| ussxh8g16bc.ibs * IBIS 4.2 Model
| 8Gb DDR3L SDRAM
| This Model is valid for Commercial Temperature Range 0C<=Tc<=85C
| Valid for DDR3L-1066/1333/1600/1866 operation
[IBIS Ver]   4.2
[File Name]   ussxh8g16bc.ibs
[Date]   10/19/2018
[File Rev]   2.0
| COMPONENT: SCB13(15)H8G162BF (96-Ball FBGA, x16, 7.5mm X 13.5mm)
[Component]   SCB13(15)H8G162BF
[Manufacturer]  UniIC Semiconductors Corp.
[Package]
|   typ   min   max
R_pkg   454.1m   301.3m   636.7m
L_pkg   1.754nH   1.047nH   2.886nH
C_pkg   0.475pF   0.334pF   0.777pF
[Pin]   signal_name  model_name   R_pin   L_pin   C_pin
A1   VDDQ   POWER
A2   DQ13   DQ
A3   DQ15   DQ
A7   DQ12   DQ
A8   VDDQ   POWER
A9   VSS   GND
B1   VSSQ   GND
B2   VDD   POWER
B3   VSS   GND
B7   UDQS#   DQS
B8   DQ14   DQ
B9   VSSQ   GND
C1   VDDQ   POWER
C2   DQ11   DQ
C3   DQ9   DQ
C7   UDQS   DQS
C8   DQ10   DQ
C9   VDDQ   POWER
D1   VSSQ   GND
D2   VDDQ   POWER
D3   UDM   DM
D7   DQ8   DQ
D8   VSSQ   GND
D9   VDD   POWER
E1   VSS   GND
E2   VSSQ   GND
E3   DQ0   DQ
E7   LDM   DM
E8   VSSQ   GND
E9   VDDQ   POWER
F1   VDDQ   POWER
F2   DQ2   DQ
F3   LDQS   DQS
F7   DQ1   DQ
F8   DQ3   DQ
F9   VSSQ   GND
G1   VSSQ   GND
G2   DQ6   DQ
G3   LDQS#   DQS
G7   VDD   POWER
G8   VSS   GND
G9   VSSQ   GND
H1   VREFDQ   POWER
H2   VDDQ   POWER
H3   DQ4   DQ
H7   DQ7   DQ
H8   DQ5   DQ
H9   VDDQ   POWER
J1   NC   NC
J2   VSS   GND
J3   RAS#   INPUT
J7   CK   CLKIN
J8   VSS   GND
J9   NC   NC
K1   ODT   INPUT
K2   VDD   POWER
K3   CAS#   INPUT
K7   CK#   CLKIN
K8   VDD   POWER
K9   CKE   INPUT
L1   NC   NC
L2   CS#   INPUT
L3   WE#   INPUT
L7   A10   INPUT
L8   ZQ   NC
L9   NC   NC
M1   VSS   GND
M2   BA0   INPUT
M3   BA2   INPUT
M7   A15   INPUT
M8   VREFCA   POWER
M9   VSS   GND
N1   VDD   POWER
N2   A3   INPUT
N3   A0   INPUT
N7   A12   INPUT
N8   BA1   INPUT
N9   VDD   POWER
P1   VSS   GND
P2   A5   INPUT
P3   A2   INPUT
P7   A1   INPUT
P8   A4   INPUT
P9   VSS   GND
R1   VDD   POWER
R2   A7   INPUT
R3   A9   INPUT
R7   A11   INPUT
R8   A6   INPUT
R9   VDD   POWER
T1   VSS   GND
T2   RESET#   RESET
T3   A13   INPUT
T7   A14   INPUT
T8   A8   INPUT
T9   VSS   GND
|***********************PIN MAPPING*****************************************
[Pin Mapping] pulldown_ref pullup_ref gnd_clamp_ref power_clamp_ref ext_ref
A1   NC   VDDQ
A2   VSS   VDDQ   VSS   VDDQ
A3   VSS   VDDQ   VSS   VDDQ
A7   VSS   VDDQ   VSS   VDDQ
A8   NC   VDDQ
A9   VSS   NC
B1   VSS   NC
B2   NC   VDD
B3   VSS   NC
B7   VSS   VDDQ   VSS   VDDQ
B8   VSS   VDDQ   VSS   VDDQ
B9   VSS   NC
C1   NC   VDDQ
C2   VSS   VDDQ   VSS   VDDQ
C3   VSS   VDDQ   VSS   VDDQ
C7   VSS   VDDQ   VSS   VDDQ
C8   VSS   VDDQ   VSS   VDDQ
C9   NC   VDDQ
D1   VSS   NC
D2   NC   VDDQ
D3   NC   NC   VSS   VDDQ
D7   VSS   VDDQ   VSS   VDDQ
D8   VSS   NC
D9   NC   VDD
E1   VSS   NC
E2   VSS   NC
E3   VSS   VDDQ   VSS   VDDQ
E7   NC   NC   VSS   VDDQ
E8   VSS   NC
E9   NC   VDDQ
F1   NC   VDDQ
F2   VSS   VDDQ   VSS   VDDQ
F3   VSS   VDDQ   VSS   VDDQ
F7   VSS   VDDQ   VSS   VDDQ
F8   VSS   VDDQ   VSS   VDDQ
F9   VSS   NC
G1   VSS   NC
G2   VSS   VDDQ   VSS   VDDQ
G3   VSS   VDDQ   VSS   VDDQ
G7   NC   VDD
G8   VSS   NC
G9   VSS   NC
H1   NC   VREFDQ
H2   NC   VDDQ
H3   VSS   VDDQ   VSS   VDDQ
H7   VSS   VDDQ   VSS   VDDQ
H8   VSS   VDDQ   VSS   VDDQ
H9   NC   VDDQ
J1   NC   NC
J2   VSSL   NC
J3   NC   NC   VSS   VDD
J7   NC   NC   VSS   VDD
J8   VSS   NC
J9   NC   NC
K1   NC   NC   VSS   VDD
K2   NC   VDDL
K3   NC   NC   VSS   VDD
K7   NC   NC   VSS   VDD
K8   NC   VDD
K9   NC   NC   VSS   VDD
L1   NC   NC
L2   NC   NC   VSS   VDD
L3   NC   NC   VSS   VDD
L7   NC   NC   VSS   VDD
L8   NC   NC
L9   NC   NC
M1   VSS   NC
M2   NC   NC   VSS   VDD
M3   NC   NC   VSS   VDD
M7   NC   NC
M8   NC   VREFCA
M9   VSS   NC
N1   NC   VDD
N2   NC   NC   VSS   VDD
N3   NC   NC   VSS   VDD
N7   NC   NC   VSS   VDD
N8   NC   NC   VSS   VDD
N9   NC   VDD
P1   VSS   NC
P2   NC   NC   VSS   VDD
P3   NC   NC   VSS   VDD
P7   NC   NC   VSS   VDD
P8   NC   NC   VSS   VDD
P9   VSS   NC
R1   NC   VDD
R2   NC   NC   VSS   VDD
R3   NC   NC   VSS   VDD
R7   NC   NC   VSS   VDD
R8   NC   NC   VSS   VDD
R9   NC   VDD
T1   VSS   NC
T2   NC   NC   VSS   VDD
T3   NC   NC   VSS   VDD
T7   NC   NC   VSS   VDD
T8   NC   NC   VSS   VDD
T9   VSS   NC
|**********************DIFF PIN*********************************************
[Diff_pin]   inv_pin   vdiff   tdelay_typ   tdelay_min   tdelay_max
   C7   B7   0.320V   0ns   NA   NA
   F3   G3   0.320V   0ns   NA   NA
   J7   K7   0.320V   0ns   NA   NA
|   Model Selector
[Model Selector] DQ
DQ_34   34 Ohm Data I/O with no ODT, 800-2133Mbps
DQ_40   40 Ohm Data I/O with no ODT, 800-2133Mbps
DQ_IN_ODT20   Data Input with 20ohm ODT, 800-2133Mbps
DQ_IN_ODT30   Data Input with 30ohm ODT, 800-2133Mbps
DQ_IN_ODT40   Data Input with 40ohm ODT, 800-2133Mbps
DQ_IN_ODT60   Data Input with 60ohm ODT, 800-2133Mbps
DQ_IN_ODT120  Data Input with 120ohm ODT, 800-2133Mbps
[Model Selector] DQS
DQS_34   34 Ohm Data Strobe I/O with no ODT, 800-2133Mbps
DQS_40   40 Ohm Data Strobe I/O with no ODT, 800-2133Mbps
DQS_IN_ODT20  Data Strobe Input with 20ohm ODT, 800-2133Mbps
DQS_IN_ODT30  Data Strobe Input with 30ohm ODT, 800-2133Mbps
DQS_IN_ODT40  Data Strobe Input with 40ohm ODT, 800-2133Mbps
DQS_IN_ODT60  Data Strobe Input with 60ohm ODT, 800-2133Mbps
DQS_IN_ODT120 Data Strobe Input with 120ohm ODT, 800-2133Mbps
[Model Selector] DM
DM_INPUT   DM Input Model with no ODT, 800-2133Mbps
DM_ODT20   DM Input Model with 20ohm ODT, 800-2133Mbps
DM_ODT30   DM Input Model with 30ohm ODT, 800-2133Mbps
DM_ODT40   DM Input Model with 40ohm ODT, 800-2133Mbps
DM_ODT60   DM Input Model with 60ohm ODT, 800-2133Mbps
DM_ODT120   DM Input Model with 120ohm ODT, 800-2133Mbps
[Model Selector] DM_TDQS
DM_INPUT   DM Input Model with no ODT, 800-2133Mbps
DM_ODT20   DM Input Model with 20ohm ODT, 800-2133Mbps
DM_ODT30   DM Input Model with 30ohm ODT, 800-2133Mbps
DM_ODT40   DM Input Model with 40ohm ODT, 800-2133Mbps
DM_ODT60   DM Input Model with 60ohm ODT, 800-2133Mbps
DM_ODT120   DM Input Model with 120ohm ODT, 800-2133Mbps
TDQS_ODT20   TDQS Terminator Model with 20ohm ODT, 800-2133Mbps
TDQS_ODT30   TDQS Terminator Model with 30ohm ODT, 800-2133Mbps
TDQS_ODT40   TDQS Terminator Model with 40ohm ODT, 800-2133Mbps
TDQS_ODT60   TDQS Terminator Model with 60ohm ODT, 800-2133Mbps
TDQS_ODT120   TDQS Terminator Model with 120ohm ODT, 800-2133Mbps
[Model Selector] NF_TDQS#
NF_INPUT   Non-Functioning Terminator Model
TDQS_ODT20   TDQS Terminator Model with 20ohm ODT, 800-2133Mbps
TDQS_ODT30   TDQS Terminator Model with 30ohm ODT, 800-2133Mbps
TDQS_ODT40   TDQS Terminator Model with 40ohm ODT, 800-2133Mbps
TDQS_ODT60   TDQS Terminator Model with 60ohm ODT, 800-2133Mbps
TDQS_ODT120   TDQS Terminator Model with 120ohm ODT, 800-2133Mbps
| Sparse Matrix Package Model for B5116ECMDXG_96ball_pkg (x16)
[Define Package Model]  KTC_8G3D_x16_RDL_DDP_PKG
[Manufacturer]  UniIC Semiconductors Corp.
[OEM]  UniIC
[Description]  None
[Number Of Pins]  51
[Pin Numbers]
|Pin Num   Terminal Name
N3   | A0:A0_DIEtop_78
P7   | A1:A1_DIEtop_83
P3   | A2:A2_DIEtop_82
N2   | A3:A3_DIEtop_74
P8   | A4:A4_DIEtop_79
P2   | A5:A5_DIEtop_80
R8   | A6:A6_DIEtop_81
R2   | A7:A7_DIEtop_84
T8   | A8:A8_DIEtop_85
R3   | A9:A9_DIEtop_86
L7   | A10:A10_DIEtop_65
R7   | A11:A11_DIEtop_87
N7   | A12:A12_DIEtop_75
T3   | A13:A13_DIEtop_88
T7   | A14:A14_DIEtop_89
M7   | A15:A15_DIEtop_73
M2   | BA0:BA0_DIEtop_70
N8   | BA1:BA1_DIEtop_71
M3   | BA2:BA2_DIEtop_72
K3   | CASB:CASB_DIEtop_62
J7   | CK:CK_DIEtop_57
K7   | CKB:CKB_DIEtop_58
K9   | CKE:CKE_DIEtop_59
L2   | CSB:CSB_DIEtop_63
E7   | DML:DML_DIEbot_30
D3   | DMU:DMU_DIEtop_30
E3   | DQL0:DQL0_DIEbot_32
F7   | DQL1:DQL1_DIEbot_34
F2   | DQL2:DQL2_DIEbot_36
F8   | DQL3:DQL3_DIEbot_38
H3   | DQL4:DQL4_DIEbot_47
H8   | DQL5:DQL5_DIEbot_45
G2   | DQL6:DQL6_DIEbot_43
H7   | DQL7:DQL7_DIEbot_49
F3   | DQSL:DQSL_DIEbot_40
G3   | DQSLB:DQSLB_DIEbot_41
C7   | DQSU:DQSU_DIEtop_40
B7   | DQSUB:DQSUB_DIEtop_41
D7   | DQU0:DQU0_DIEtop_32
C3   | DQU1:DQU1_DIEtop_34
C8   | DQU2:DQU2_DIEtop_36
C2   | DQU3:DQU3_DIEtop_38
A7   | DQU4:DQU4_DIEtop_47
A2   | DQU5:DQU5_DIEtop_45
B8   | DQU6:DQU6_DIEtop_43
A3   | DQU7:DQU7_DIEtop_49
J1   | ODT:ODT_DIEtop_61
J3   | RASB:RASB_DIEtop_60
T2   | RESETB:RESETB_DIEtop_92
L3   | WEB:WEB_DIEtop_64
L8   | ZQ:ZQ_DIEtop_69
[Model Data]
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[End Model Data]
[End Package Model]
| Models and submodels in the file (29): DQ_34 (I/O), DQ_40 (I/O), DQ_IN_ODT20 (Input), DQ_IN_ODT30 (Input), DQ_IN_ODT40 (Input), DQ_IN_ODT60 (Input), DQ_IN_ODT120 (Input), DQS_34 (I/O), DQS_40 (I/O), DQS_IN_ODT20 (Input), DQS_IN_ODT30 (Input), DQS_IN_ODT40 (Input), DQS_IN_ODT60 (Input), DQS_IN_ODT120 (Input), DM_INPUT (Input), DM_ODT20 (Input), DM_ODT30 (Input), DM_ODT40 (Input), DM_ODT60 (Input), DM_ODT120 (Input), TDQS_ODT20 (Terminator), TDQS_ODT30 (Terminator), TDQS_ODT40 (Terminator), TDQS_ODT60 (Terminator), TDQS_ODT120 (Terminator), INPUT (Input), CLKIN (Input), RESET (Input), NF_INPUT (Terminator)
